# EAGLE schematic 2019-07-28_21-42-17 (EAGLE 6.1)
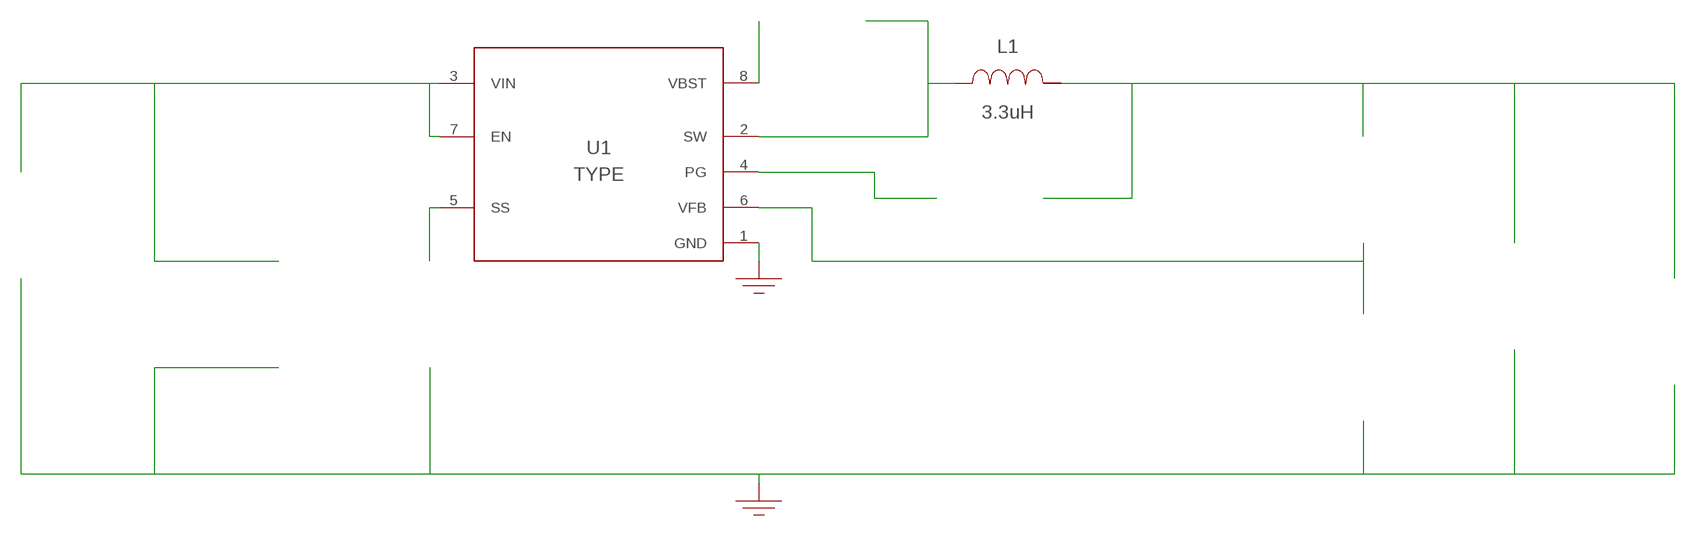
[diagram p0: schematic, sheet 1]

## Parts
CBST  100nF  C0603C104Z3VACTUC0603C104Z3VACTU  [0603]  (not placed on a sheet)
CIN  10uF  GRM31CR61E106KA12LGRM31CR61E106KA12L  [1206_190]  (not placed on a sheet)
CIN_2  10uF  GRM31CR61E106KA12LGRM31CR61E106KA12L  [1206_190]  (not placed on a sheet)
COUT  47uF  C3216X5R1E476M160ACC3216X5R1E476M160AC  [1206]  (not placed on a sheet)
CSS  8.2nF  GRM033R71A822KA01DGRM033R71A822KA01D  [0201]  (not placed on a sheet)
GND  WB_GND  WB_GNDWB_GND  [WB_GND]
GND2  WB_GND  WB_GNDWB_GND  [WB_GND]
IOUT  WB_CURRENT_LOAD  WB_CURRENT_LOADWB_CURRENT_LOAD  [WB_CURRENT_LOAD]  (not placed on a sheet)
L1  3.3uH  VLP8040T-3R3NVLP8040T-3R3N  [VLP8040]
RFBB  10k  RC0201FR-0710KLRC0201FR-0710KL  [0201]  (not placed on a sheet)
RFBT  56.2k  RC0201FR-0756K2LRC0201FR-0756K2L  [0201]  (not placed on a sheet)
RPG  100k  CRCW0402100KFKEDCRCW0402100KFKED  [0402]  (not placed on a sheet)
U1  TPS563210ADDFR  TPS563210ADDFRTPS563210ADDFR  [DDF0008A_N]
VIN  WB_BATTERY  WB_BATTERYWB_BATTERY  [WB_BATTERY]  (not placed on a sheet)

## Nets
0: Cin.2@2 Cin_2.2@2 Cout.2@2 Css.2@2 GND2.1 GND.1 Iout.-@2 Rfbb.2@2 U1.1(GND) Vin.-@2
1: Rpg.2@2 U1.4(PG)
2: Rfbb.1@1 Rfbt.2@2 U1.6(VFB)
3: Cin.1@1 Cin_2.1@1 U1.3(VIN) U1.7(EN) Vin.+@1
4: Cout.1@1 Iout.+@1 L1.2 Rfbt.1@1 Rpg.1@1
5: Cbst.1@1 L1.1 U1.2(SW)
6: Css.1@1 U1.5(SS)
7: Cbst.2@2 U1.8(VBST)
Unconnected: CBST.1 CBST.2 CIN.1 CIN.2 CIN_2.1 CIN_2.2 COUT.1 COUT.2 CSS.1 CSS.2 IOUT.1(+) IOUT.2(-) RFBB.1 RFBB.2 RFBT.1 RFBT.2 RPG.1 RPG.2 VIN.1(+) VIN.2(-)

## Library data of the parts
CBST = AcceleratedDesigns_Lib:C0603C104Z3VACTU; Cap: 1.0E-7; ESR: 0.0; IRMS: 0.0; Manufacturer_Name: Kemet; Manufacturer_Part_Number: C0603C104Z3VACTU; VDC: 25.0; Vendor: Kemet
CIN CIN_2 = AcceleratedDesigns_Lib:GRM31CR61E106KA12L; Cap_F: 0.00001; ESR_ohm: 0.004; Manufacturer_Name: MuRata; Manufacturer_Part_Number: GRM31CR61E106KA12L; Technology: Ceramic; VDC_V: 25
COUT = AcceleratedDesigns_Lib:C3216X5R1E476M160AC; Cap_F: 0.000047; Manufacturer_Name: TDK; Manufacturer_Part_Number: C3216X5R1E476M160AC; MountType: SMT; RoHS: Y; VDC_V: 25
CSS = AcceleratedDesigns_Lib:GRM033R71A822KA01D; Cap: 8.2E-9; ESR: 0.0; IRMS: 0.0; Manufacturer_Name: MuRata; Manufacturer_Part_Number: GRM033R71A822KA01D; VDC: 10.0; Vendor: MuRata
GND GND2 = AcceleratedDesigns_Lib:WB_GND; Manufacturer_Name: WB_GND; Manufacturer_Part_Number: WB_GND; PowerPortType: POWER_GROUND; Value: Value
IOUT = AcceleratedDesigns_Lib:WB_CURRENT_LOAD; Manufacturer_Name: WB_CURRENT_LOAD; Manufacturer_Part_Number: WB_CURRENT_LOAD; PowerPortType: POWER_GROUND; Value: Value
L1 = AcceleratedDesigns_Lib:VLP8040T-3R3N; DCR: 0.02; Datasheet_URL: http://www.tdk.co.jp/tjfx01/j531_vlp.pdf; Description: Unknown; IDC: 5.2; L: 3.3E-6; Manufacturer: TDK; Manufacturer_Name: TDK; Manufacturer_Part_Number: VLP8040T-3R3N; PACKAGE_DESIGNATOR: VLP8040; Vendor: TDK
RFBB = AcceleratedDesigns_Lib:RC0201FR-0710KL; Datasheet_URL: http://www.yageo.com/documents/recent/PYu%2DRC%5FGroup%5F51%5FRoHS%5FL%5F5.pdf; Manufacturer_Name: Yageo; Manufacturer_Part_Number: RC0201FR-0710KL; Power: 0.05; Resistance: 10000.0; Tolerance: 1.0; Vendor: Yageo America
RFBT = AcceleratedDesigns_Lib:RC0201FR-0756K2L; Datasheet_URL: http://www.yageo.com/documents/recent/PYu%2DRC%5FGroup%5F51%5FRoHS%5FL%5F5.pdf; Manufacturer_Name: Yageo; Manufacturer_Part_Number: RC0201FR-0756K2L; Power: 0.05; Resistance: 56200.0; Tolerance: 1.0; Vendor: Yageo America
RPG = AcceleratedDesigns_Lib:CRCW0402100KFKED; Manufacturer_Name: Vishay-Dale; Manufacturer_Part_Number: CRCW0402100KFKED; Power: 0.063; Resistance: 100000.0; Tolerance: 1.0; Vendor: Vishay-Dale
U1 = AcceleratedDesigns_Lib:TPS563210ADDFR; Manufacturer: Texas Instruments; Manufacturer_Name: Texas Instruments; Manufacturer_Part_Number: TPS563210ADDFR; PartNumber: TPS563210ADDFR; RefDes: RefDes; TYPE: TYPE; Value: Value
VIN = AcceleratedDesigns_Lib:WB_BATTERY; Manufacturer_Name: WB_BATTERY; Manufacturer_Part_Number: WB_BATTERY; PowerPortType: POWER_GROUND; Value: Value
